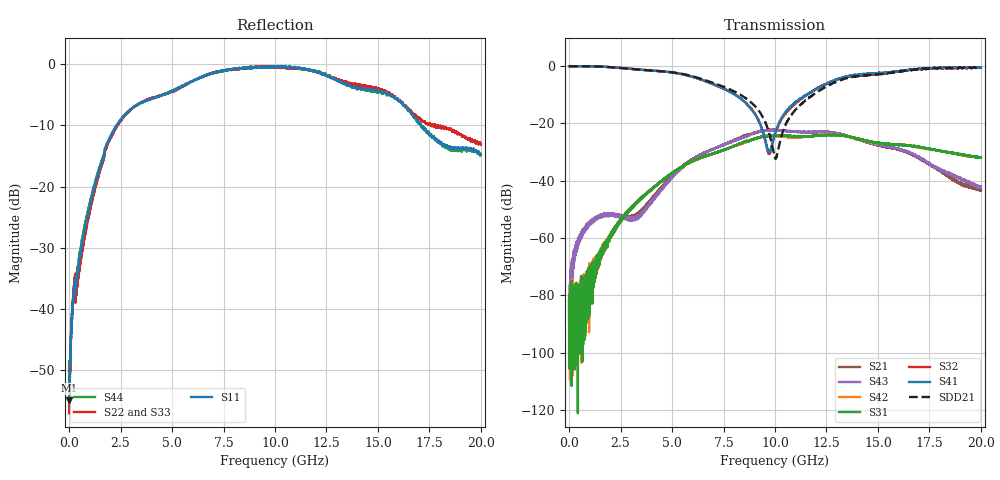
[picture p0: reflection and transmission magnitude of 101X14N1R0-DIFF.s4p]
!{X14N1R0}
!Johanson Technology Inc.
!www.johansontechnology.com
!Test Board Conditions:
!Substrate Type  RO4350B
!Substrate Thickness  10 mil
!Substrate Dk  3.66
!TL Type: GCPW
!TL Trace Width  20 mil
!TL Gap  15 mil
!PART MODE DIFFERENTIAL
!DUT TOPOLOGY	DIFFERENTIAL 4-PORT
!Mounting Pad LxW  20x35 mil
# MHz S  dB  R 50
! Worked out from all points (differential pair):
!   20001 points, 300 kHz to 20 GHz, reference 50 ohm
!   strongest paths, dB at 300 kHz, 5 GHz, 10 GHz, 15 GHz, 20 GHz:
!     S41: 0.0, -2.2, -23.5, -2.4, -0.5
!     S32: 0.0, -2.2, -23.8, -2.8, -0.5
!     S31: -89.6, -37.3, -24.1, -26.8, -32.0
!     S42: -81.7, -37.4, -24.4, -27.0, -32.0
!     S43: -83.0, -38.8, -22.4, -27.3, -42.0
!     S21: -81.7, -38.3, -22.2, -27.6, -43.2
!   taken as a pair (ports 1,2 in; 4,3 out), SDD21 dB: 0.0, -2.1, -32.0, -2.9, -0.5
!   lowest |S11| = -55.0 dB at 3.3 MHz (marker M1), VSWR 1.00, Z = 50.2 - j0.0185 ohm
!   |S11| at or under -10 dB: start of sweep to 2.304 GHz; 17.1 GHz to end of sweep
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0.3  -51.29 -12.2  -78.04 -149.9  -83.26 132.7  -0.02 -0.1
     -81.73 87.3  -57.12 168.6  0.01 0.1  -81.49 27.6
     -89.64 -86.2  0.01 0.2  -58.60 -163.2  -88.21 -62.2
     -0.03 -0.1  -81.69 -117.7  -83.04 96.1  -48.57 -9.3
3.3  -54.96 -5.9  -90.65 -42.7  -95.69 148.5  -0.02 -0.0
     -84.60 102.7  -56.19 -4.5  -0.02 0.0  -88.84 -85.0
     -98.61 -33.9  -0.02 0.0  -56.26 -10.5  -84.37 144.1
     -0.01 -0.0  -90.40 123.2  -86.44 84.0  -54.57 -7.4
954.286  -23.96 -102.8  -55.39 78.8  -76.12 -44.1  -0.04 -11.2
         -55.37 77.5  -24.83 -101.5  -0.04 -11.7  -75.73 -54.8
         -70.25 -57.1  -0.04 -11.7  -24.43 -103.0  -55.36 77.9
         -0.05 -11.1  -77.16 -73.2  -55.26 75.7  -23.40 -101.7
3425.249  -6.39 -130.2  -51.16 120.9  -46.49 -127.0  -1.17 -39.8
          -51.10 123.4  -6.32 -131.4  -1.20 -40.5  -46.43 -126.4
          -46.70 -126.7  -1.20 -40.6  -6.35 -129.6  -52.06 121.6
          -1.17 -39.8  -46.51 -125.8  -52.44 121.1  -6.45 -129.6
9713.154  -0.33 130.8  -22.23 39.1  -24.27 44.5  -29.93 -46.2
          -22.21 39.4  -0.41 128.8  -30.62 -45.5  -24.34 45.4
          -24.22 44.1  -30.62 -45.8  -0.46 139.3  -22.35 50.6
          -29.93 -46.3  -24.38 45.1  -22.42 51.0  -0.44 143.3
12613.11  -1.96 90.9  -23.04 -26.7  -24.01 -35.1  -5.72 3.2
          -23.01 -27.2  -1.97 93.1  -5.62 1.3  -23.81 -32.8
          -23.96 -34.8  -5.68 1.7  -1.69 101.9  -22.94 -14.7
          -5.72 3.4  -23.88 -31.8  -22.93 -14.7  -1.77 105.8
20000  -14.82 10.0  -43.35 -128.1  -31.92 -170.3  -0.44 -80.9
       -43.20 -130.2  -13.09 4.0  -0.48 -81.3  -31.90 -170.1
       -31.96 -170.5  -0.48 -81.1  -12.97 18.5  -42.42 -111.9
       -0.46 -80.7  -31.96 -169.8  -42.00 -111.9  -14.69 14.2
